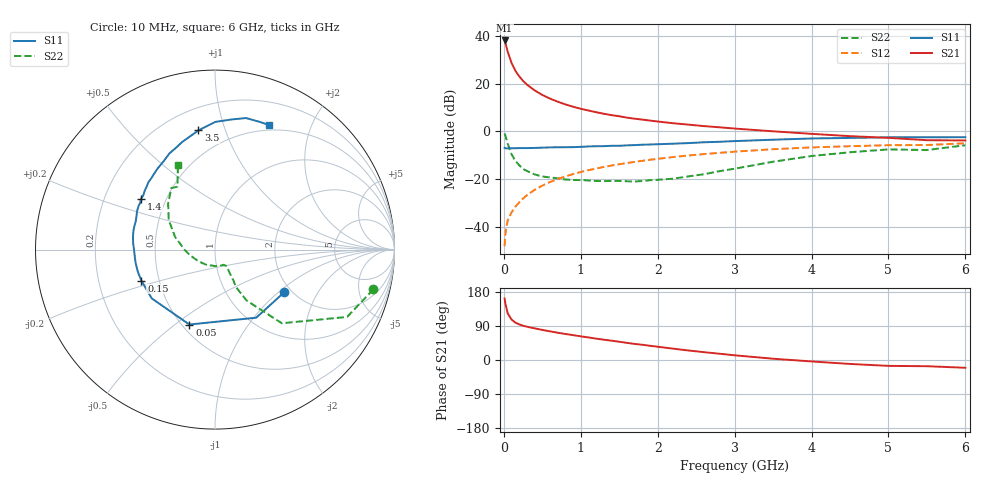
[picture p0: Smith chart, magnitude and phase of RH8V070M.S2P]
! SIEMENS Small Signal Semiconductors
! BFR106
! Si NPN RF Bipolar Junction Transistor in SOT23
! VCE = 8 V  IC = 70 mA
! Common Emitter S-Parameters:  August  1996
# GHz  S  MA  R  50
!  f  S11  S21  S12  S22
! GHz  MAG  ANG  MAG  ANG  MAG  ANG  MAG  ANG
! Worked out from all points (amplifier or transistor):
!   36 points, 10 MHz to 6 GHz, reference 50 ohm
!   highest |S21| = 38.0 dB at 10 MHz (marker M1)
!   |S21| within 3 dB of that: start of sweep to 36.48 MHz
!   unconditionally stable (mu >= 1): 222.2 MHz to 2.341 GHz
!   at 250 MHz: K = 1.02, MAG = 23.6 dB, |S12| = -28.0 dB
!   at 1.4 GHz: K = 1.06, MAG = 9.0 dB, |S12| = -14.3 dB
!   at 6 GHz: K = 0.98, MSG = 0.6 dB, |S12| = -5.0 dB
!   S11 on the Smith chart (normalised r, x): 10 MHz: 1.83, -1.10; 50 MHz: 0.54, -0.56; 150 MHz: 0.40, -0.17; 1.4 GHz: 0.36, +0.27; 3.5 GHz: 0.34, +0.81; 6 GHz: 0.44, +1.43
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0.01  0.4532 -31.6  79.47 162.4  0.004 79.5  0.9098 -14.1
0.02  0.4435 -58.8  71.3 148.8  0.0073 69.1  0.8261 -27.0
0.05  0.4412 -108.9  46.32 123.4  0.0138 61.7  0.554 -47.8
0.1  0.445 -142.3  26.98 106.7  0.0202 61.1  0.3331 -58.2
0.15  0.4451 -157.1  18.54 98.6  0.0267 66.1  0.2418 -60.7
0.2  0.4474 -164.2  14.15 94.1  0.0329 68.2  0.1966 -59.1
0.25  0.4483 -170.2  11.35 90.4  0.0396 69.4  0.1644 -58.3
0.3  0.4484 -173.8  9.5 87.9  0.0464 71.4  0.1492 -57.8
0.4  0.4514 179.9  7.198 83.5  0.0601 72.2  0.1263 -55.7
0.5  0.4579 175.2  5.774 79.4  0.0734 72.4  0.1142 -54.7
0.6  0.4629 170.8  4.843 75.6  0.0874 72.0  0.1091 -55.6
0.7  0.4662 167.2  4.18 72.0  0.1013 71.0  0.1047 -57.9
0.9  0.4687 160.5  3.279 65.6  0.1283 69.1  0.0965 -61.2
1.1  0.4844 153.7  2.732 59.5  0.1547 66.8  0.0944 -70.2
1.4  0.5006 145.5  2.187 51.0  0.1934 62.7  0.0922 -83.1
1.7  0.5174 137.4  1.843 42.4  0.2306 58.7  0.09 -100.8
2.2  0.5539 125.2  1.482 30.0  0.2909 51.6  0.1029 -132.8
2.8  0.6067 111.2  1.219 16.6  0.3565 42.7  0.1473 -170.2
3.5  0.6706 97.9  1.005 3.4  0.4247 32.5  0.2325 162.6
4.5  0.7307 82.8  0.796 -10.4  0.4902 17.9  0.3668 135.4
5.5  0.7542 70.4  0.655 -16.4  0.5205 7.8  0.4081 120.8
6  0.7563 66.4  0.646 -20.5  0.5646 0.9  0.5144 113.7
